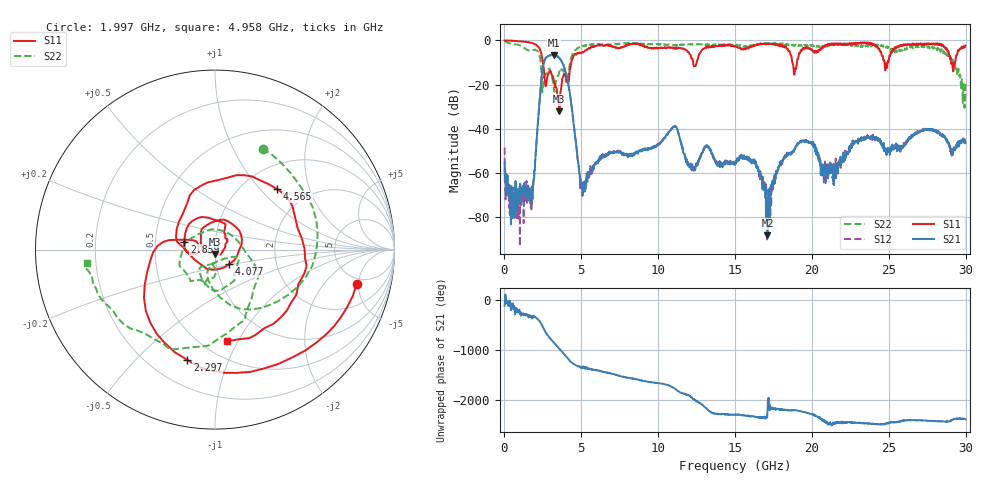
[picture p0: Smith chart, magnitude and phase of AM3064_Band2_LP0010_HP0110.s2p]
# Hz S DB R 50.0
!freq dBS11 angS11 dBS21 angS21 dBS12 angS12 dBS22 angS22
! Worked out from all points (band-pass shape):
!   1600 points, 10 MHz to 29.98 GHz, reference 50 ohm
!   highest |S21| = -6.57 dB at 3.234 GHz (marker M1); lowest = -88.1 dB at 17.1 GHz (marker M2)
!   |S21| within 3 dB of the highest: 2.579 GHz to 3.725 GHz (1.145 GHz wide, 36.3 % of centre)
!   lowest |S11| = -32.1 dB at 3.571 GHz (marker M3), VSWR 1.05, Z = 50.1 - j2.5 ohm
!   |S11| at or under -10 dB: 2.506 GHz to 4.348 GHz (1.842 GHz wide, 53.7 % of centre); 12.27 GHz to 12.49 GHz (228.3 MHz wide, 1.84 % of centre); 18.73 GHz to 19.02 GHz (291.9 MHz wide, 1.55 % of centre)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
!   |S22| runs from -30.5 to -0.3 dB; largest |S21 - S12| = 0.013
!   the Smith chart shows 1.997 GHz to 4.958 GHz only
!   S11 on the Smith chart (normalised r, x): 1.997 GHz: 4.24, -4.73; 2.297 GHz: 0.35, -0.72; 2.859 GHz: 0.71, +0.06; 4.077 GHz: 1.16, -0.19; 4.565 GHz: 1.42, +1.25; 4.958 GHz: 0.65, -0.90
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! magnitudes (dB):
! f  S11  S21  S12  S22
! 10 MHz  0.0  -55.0  -48.5  -0.3
! 778.5 MHz  -0.3  -78.2  -68.3  -1.8
! 1.734 GHz  -1.1  -69.0  -72.0  -4.6
! 1.997 GHz  -1.8  -54.6  -53.7  -4.2
! 2.297 GHz  -4.0  -26.1  -26.0  -7.5
! 2.859 GHz  -15.1  -7.0  -7.0  -13.2
! 3.234 GHz  -19.0  -6.6  -6.6  -22.7
! 3.571 GHz  -32.1  -8.0  -8.0  -14.1
! 4.077 GHz  -18.9  -17.0  -17.0  -19.0
! 4.565 GHz  -6.3  -41.4  -41.5  -4.5
! 4.958 GHz  -5.8  -63.7  -65.4  -2.9
! 5.015 GHz  -5.7  -65.3  -64.1  -2.9
! 10 GHz  -3.5  -46.8  -46.7  -1.8
! 15 GHz  -2.6  -55.5  -56.3  -1.9
! 16.32 GHz  -2.2  -55.1  -55.2  -2.0
! 17.1 GHz  -1.5  -88.1  -73.8  -1.4
! 18.27 GHz  -3.1  -52.8  -51.7  -2.0
! 19.99 GHz  -4.1  -46.4  -46.8  -2.0
! 20.78 GHz  -2.6  -64.2  -63.4  -3.0
! 25 GHz  -9.0  -50.5  -48.4  -2.9
! 28.56 GHz  -2.6  -43.3  -43.2  -4.7
! 29.98 GHz  -2.4  -46.2  -46.8  -19.2
